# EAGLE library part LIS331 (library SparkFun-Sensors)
ST Microelectronics LIS331 3-Axis &plusmn;6/12/24g SPI/I2C Accelerometer The LIS331HH is an ultra low-power full-scale three axis MEMS linear accelerometer. It has a digital I2C/SPI serial interface which makes it ideal for using in embedded applications. The device also features ultra low-power operational modes that allow advanced power saving and smart sleep to wake-up functions. Datasheet SparkFun Products SparkFun Triple Axis Accelerometer Breakout - LIS331 (SEN-10345) Triple Axis Accelerometer - LIS331HH (SEN-09755)
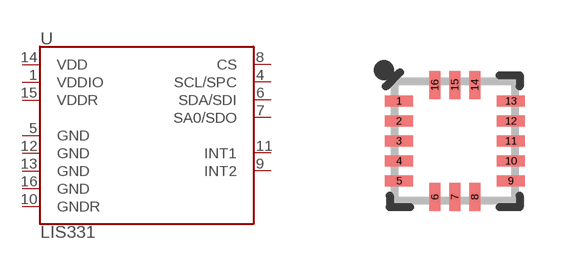
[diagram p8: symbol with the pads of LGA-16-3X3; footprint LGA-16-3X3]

Designator prefix U

## LIS331 (PROD_ID: IC-12675; SF_ID: COM-09755)  [LGA-16-3X3]
1  VDDIO
4  SCL/SPC
5  GND
6  SDA/SDI
7  SA0/SDO
8  CS
9  INT2
10  GNDR
11  INT1
12  GND
13  GND
14  VDD
15  VDDR
16  GND

## Footprint LGA-16-3X3 (pad centres in mm)
16-Pin Land Grid Array (LGA) (3 x 3 mm) Datasheet Specifications: Pin Count: 16 Area: 3.0 x 3.0 x 1.0 mm Pitch: 0.5 mm Devices Using: LIS331 LIS3DH
smd 0.7 x 0.28: 1 -1.4,1; 2 -1.4,0.5; 3 -1.4,0; 4 -1.4,-0.5; 5 -1.4,-1; 9 1.4,-1; 10 1.4,-0.5; 11 1.4,0; 12 1.4,0.5; 13 1.4,1
smd 0.28 x 0.7: 6 -0.5,-1.4; 7 0,-1.4; 8 0.5,-1.4; 14 0.5,1.4; 15 0,1.4; 16 -0.5,1.4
